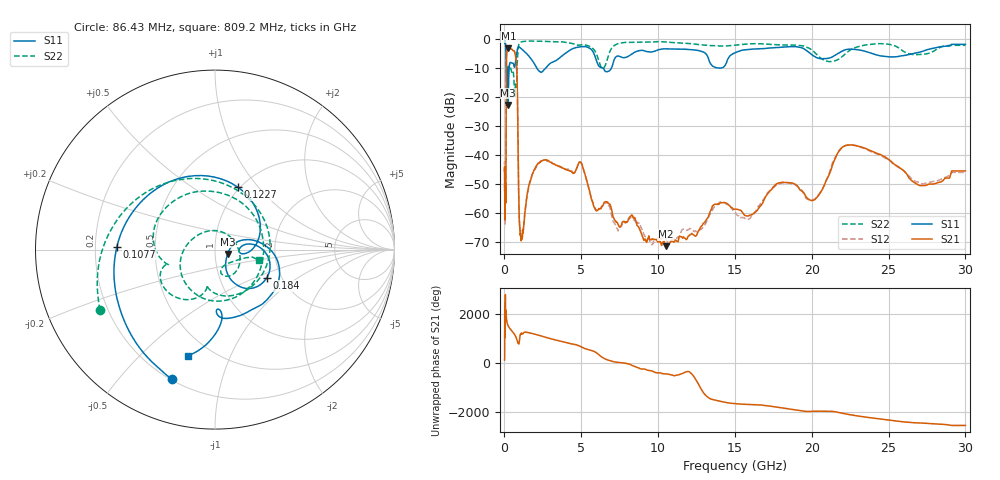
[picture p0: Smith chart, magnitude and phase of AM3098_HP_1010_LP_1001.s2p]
! Date/Time: Thu, Feb 28, 2019 8:42 AM
! Network Analyzer: Agilent Technologies E8364B Rev: A.07.50.67
! Sweep from 0.010 to 30.000 GHz, 1601 Points, Sweep Type: LOG
! Power Supply: 5.023 V, 0.002 A
# Hz S DB R 50
!freq MagS11 AngS11 MagS21 AngS21 MagS12 AngS12 MagS22 AngS22
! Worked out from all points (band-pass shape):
!   1601 points, 10 MHz to 30 GHz, reference 50 ohm
!   highest |S21| = -3.06 dB at 257.3 MHz (marker M1); lowest = -71.3 dB at 10.49 GHz (marker M2)
!   |S21| within 3 dB of the highest: 133.9 MHz to 735.8 MHz (601.9 MHz wide, 138 % of centre)
!   lowest |S11| = -22.6 dB at 241.1 MHz (marker M3), VSWR 1.16, Z = 57.5 - j2.76 ohm
!   |S11| at or under -10 dB: 191.6 MHz to 304.7 MHz (113.1 MHz wide, 45.6 % of centre); 2.118 GHz to 2.668 GHz (550.1 MHz wide, 23 % of centre); 6.433 GHz to 6.951 GHz (517.8 MHz wide, 7.74 % of centre)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
!   |S22| runs from -19.8 to -0.5 dB; largest |S21 - S12| = 0.012
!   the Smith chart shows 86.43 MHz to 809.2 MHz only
!   S11 on the Smith chart (normalised r, x): 86.43 MHz: 0.20, -0.70; 107.7 MHz: 0.29, +0.01; 122.7 MHz: 0.98, +0.79; 184 MHz: 1.68, -0.59; 809.2 MHz: 0.38, -0.71
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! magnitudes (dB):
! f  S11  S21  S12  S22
! 10 MHz  -0.3  -45.3  -46.2  -0.6
! 38.04 MHz  -0.4  -60.2  -60.7  -0.9
! 48.13 MHz  -0.7  -49.1  -49.8  -1.3
! 86.43 MHz  -2.4  -55.1  -55.3  -2.8
! 107.7 MHz  -5.2  -31.2  -31.3  -6.6
! 122.7 MHz  -8.6  -11.6  -11.6  -10.4
! 144.7 MHz  -17.5  -4.6  -4.6  -13.6
! 184 MHz  -9.7  -3.7  -3.7  -9.0
! 241.1 MHz  -22.6  -3.1  -3.0  -11.3
! 257.3 MHz  -18.2  -3.1  -3.0  -11.0
! 550.5 MHz  -8.2  -3.8  -3.8  -10.8
! 809.2 MHz  -4.3  -11.8  -11.8  -11.9
! 954.5 MHz  -2.6  -60.6  -61.2  -1.5
! 1.05 GHz  -3.0  -67.5  -67.3  -1.0
! 2.084 GHz  -9.7  -43.5  -43.8  -0.6
! 4.952 GHz  -2.5  -42.3  -42.3  -1.9
! 6.391 GHz  -9.8  -57.4  -56.8  -10.0
! 7.926 GHz  -6.1  -62.8  -63.1  -1.0
! 10.49 GHz  -3.3  -71.3  -68.3  -0.9
! 20.1 GHz  -5.6  -55.5  -55.2  -4.0
! 22.56 GHz  -3.3  -36.4  -36.4  -3.5
! 30 GHz  -1.7  -45.3  -45.8  -2.0
